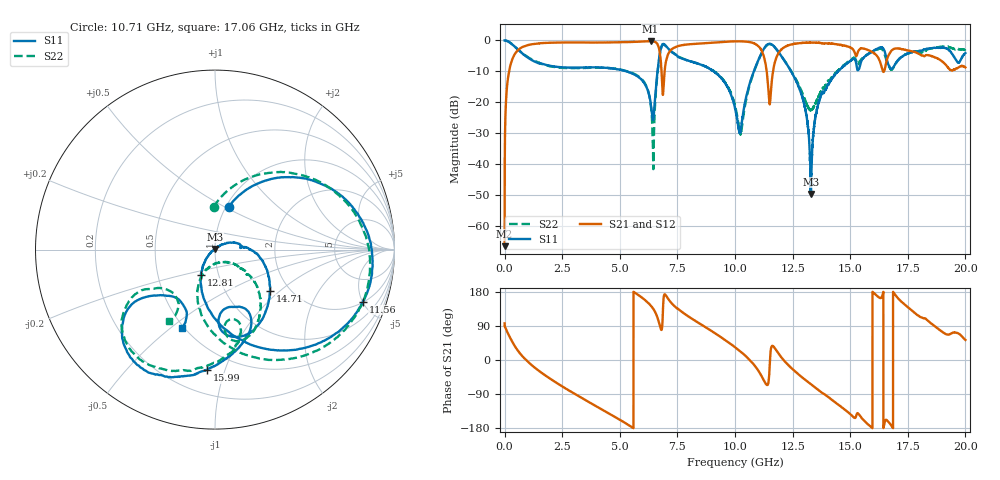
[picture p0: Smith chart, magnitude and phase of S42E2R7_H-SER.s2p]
! Created Wed Nov 25 21:41:09 2020
# khz S ma R 50
! 2 Port Network Data from SP1.SP block
! freq  magS11  angS11  magS21  angS21  magS12  angS12  magS22  angS22
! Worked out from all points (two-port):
!   20001 points, 300 kHz to 20 GHz, reference 50 ohm
!   highest |S21| = -0.23 dB at 6.333 GHz (marker M1); lowest = -66.4 dB at 300 kHz (marker M2)
!   |S21| within 3 dB of the highest: 567.1 MHz to 6.721 GHz (6.154 GHz wide, 169 % of centre); 7.198 GHz to 11.15 GHz (3.953 GHz wide, 43.1 % of centre)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
!   lowest |S11| = -49.6 dB at 13.3 GHz (marker M3), VSWR 1.01, Z = 49.8 + j0.286 ohm
!   |S11| at or under -10 dB: 5.299 GHz to 6.637 GHz (1.338 GHz wide, 22.4 % of centre); 9.081 GHz to 10.82 GHz (1.735 GHz wide, 17.4 % of centre); 12.43 GHz to 14.47 GHz (2.031 GHz wide, 15.1 % of centre)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
!   |S22| runs from -41.6 to 0.0 dB; largest |S21 - S12| = 0.016
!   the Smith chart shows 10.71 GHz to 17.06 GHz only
!   S11 on the Smith chart (normalised r, x): 10.71 GHz: 1.03, +0.52; 11.56 GHz: 2.06, -5.04; 12.81 GHz: 0.82, -0.24; 14.71 GHz: 1.60, -0.86; 15.99 GHz: 0.36, -0.87; 17.06 GHz: 0.49, -0.55
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300  0.9999 -0.2  0.0004759 96.6  0.0004924 82.0  1 -0.3
123300  0.9758 -16.7  0.2096 73.0  0.2104 73.0  0.9768 -16.6
424300  0.8052 -51.8  0.586 38.5  0.5879 38.5  0.8069 -51.8
1369300  0.444 -113.3  0.8851 -23.0  0.8847 -23.1  0.4571 -113.4
3334300  0.3654 166.6  0.9283 -99.7  0.9281 -99.7  0.3594 173.3
6333300  0.101 80.9  0.9736 144.4  0.9714 144.3  0.09931 50.6
6475300  0.06232 161.2  0.9622 132.8  0.9619 132.8  0.02281 -169.9
6667300  0.3964 -178.9  0.8213 105.9  0.8226 105.8  0.3773 -179.6
6965300  0.8443 100.6  0.3718 173.0  0.3729 172.8  0.8361 92.8
8369300  0.4249 8.7  0.8881 99.8  0.8843 99.9  0.4243 9.7
1.00003e7  0.08076 -42.0  0.967 33.8  0.9676 33.9  0.08827 -71.1
1.07133e7  0.2467 72.2  0.9275 -4.8  0.9263 -4.6  0.2372 91.9
1.15613e7  0.8735 -19.4  0.1543 30.3  0.155 30.7  0.8655 -25.1
1.28123e7  0.1605 -119.0  0.9059 -40.8  0.9076 -41.2  0.1744 -116.6
1.32973e7  0.003305 119.9  0.925 -64.2  0.9224 -64.1  0.07558 -75.9
1.33343e7  0.011 57.5  0.92 -66.0  0.921 -65.9  0.07666 -67.7
1.37073e7  0.1217 17.9  0.9116 -83.4  0.9109 -83.2  0.1452 -36.1
1.47073e7  0.382 -36.7  0.8329 -128.2  0.8305 -128.2  0.3921 -49.6
1.59853e7  0.6708 -93.9  0.641 179.0  0.6428 179.0  0.6619 -96.8
1.66673e7  0.4007 -140.6  0.5781 -164.0  0.5685 -163.7  0.3878 -146.3
1.70623e7  0.4734 -113.0  0.7424 163.9  0.7301 164.0  0.4716 -122.7
2e7  0.6265 151.1  0.3664 53.0  0.3685 53.6  0.6836 111.8
